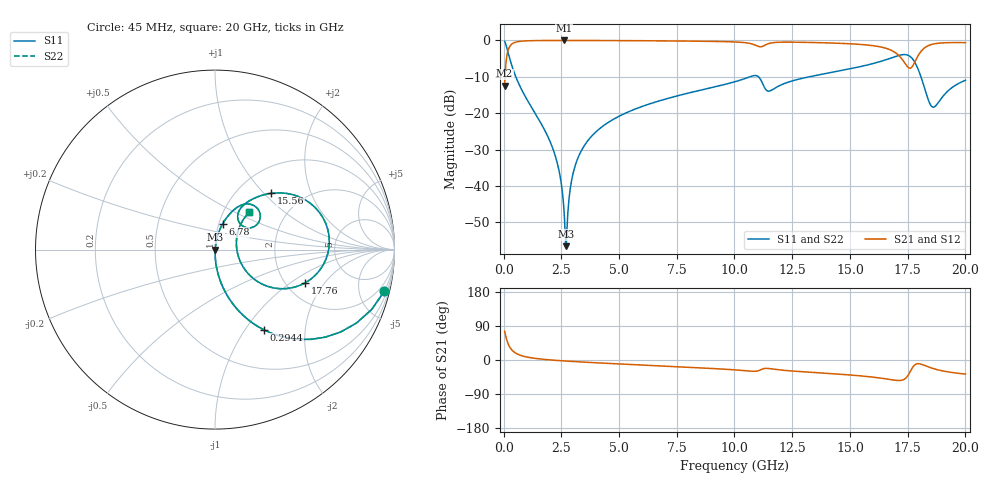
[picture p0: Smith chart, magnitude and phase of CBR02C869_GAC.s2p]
! S-parameter model data by Modelithics Inc.  support@modelithics.com 813-866-6335  Tampa FL USA
! S-Parameter data specifications:
! Substrate: 20-mil Rogers 4350B, substrate thickness, H=0.508mm, Dielectric constant, Er=3.75
! PCB Mounting Pad Footprint: Pad width, PadW=0.32mm , Pad length, PadL=0.37mm , Pad gap, PadG (edge-to-edge)=0.19mm , Reference planes=0.93mm apart
#  GHz  S  MA  R 50
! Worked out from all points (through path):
!   801 points, 45 MHz to 20 GHz, reference 50 ohm
!   highest |S21| = -0.01 dB at 2.614 GHz (marker M1); lowest = -12.5 dB at 45 MHz (marker M2)
!   group delay of S21, straight-line fit = 7.05 ps
!   lowest |S11| = -56.6 dB at 2.714 GHz (marker M3), VSWR 1.00, Z = 50.1 + j0.048 ohm
!   |S11| at or under -10 dB: 530 MHz to 10.67 GHz (10.14 GHz wide, 181 % of centre); 11.04 GHz to 13.24 GHz (2.195 GHz wide, 18.1 % of centre); 18.08 GHz to end of sweep
!   |S22| runs from -56.6 to -0.3 dB; largest |S21 - S12| = 0
!   S11 on the Smith chart (normalised r, x): 45 MHz: 0.99, -8.14; 294.4 MHz: 0.99, -1.23; 6.78 GHz: 1.04, +0.30; 15.56 GHz: 1.41, +1.10; 17.76 GHz: 2.51, -1.31; 20 GHz: 1.32, +0.60
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0.045  0.9713 -13.8  0.2379 76.2  0.2379 76.2  0.9713 -13.8
0.294438  0.5248 -58.6  0.8506 31.3  0.8506 31.3  0.5248 -58.6
0.743425  0.2227 -77.7  0.974 12.1  0.974 12.1  0.2227 -77.7
2.140275  0.03215 -88.1  0.9982 -0.4  0.9982 -0.4  0.03215 -88.1
2.4396  0.0141 -86.3  0.9985 -1.7  0.9985 -1.7  0.0141 -86.3
2.614206  0.004772 -75.9  0.9986 -2.5  0.9986 -2.5  0.004772 -75.9
2.713981  0.001486 18.8  0.9986 -2.8  0.9986 -2.8  0.001486 18.8
2.988363  0.01384 80.2  0.9984 -3.9  0.9984 -3.9  0.01384 80.2
3.387462  0.03127 81.9  0.9979 -5.3  0.9979 -5.3  0.03127 81.9
4.559819  0.0756 79.6  0.9953 -9.1  0.9953 -9.1  0.0756 79.6
6.704981  0.1464 73.8  0.9869 -15.4  0.9869 -15.4  0.1464 73.8
6.779813  0.1488 73.6  0.9865 -15.6  0.9865 -15.6  0.1488 73.6
10.0225  0.2706 61.7  0.9523 -26.1  0.9523 -26.1  0.2706 61.7
10.94542  0.3282 42.6  0.8493 -29.5  0.8493 -29.5  0.3282 42.6
11.49418  0.2008 45.3  0.9068 -22.6  0.9068 -22.6  0.2008 45.3
13.36496  0.3224 55.6  0.9363 -32.6  0.9363 -32.6  0.3224 55.6
15.56001  0.4442 44.9  0.8754 -42.5  0.8754 -42.5  0.4442 44.9
16.68248  0.559 31.2  0.7558 -50.9  0.7558 -50.9  0.559 31.2
17.38091  0.6393 5.6  0.4864 -49.7  0.4864 -49.7  0.6393 5.6
17.75506  0.5337 -20.4  0.4667 -16.1  0.4667 -16.1  0.5337 -20.4
18.57821  0.1214 1.1  0.8869 -22.0  0.8869 -22.0  0.1214 1.1
20  0.2832 47.3  0.9315 -37.1  0.9315 -37.1  0.2832 47.3
